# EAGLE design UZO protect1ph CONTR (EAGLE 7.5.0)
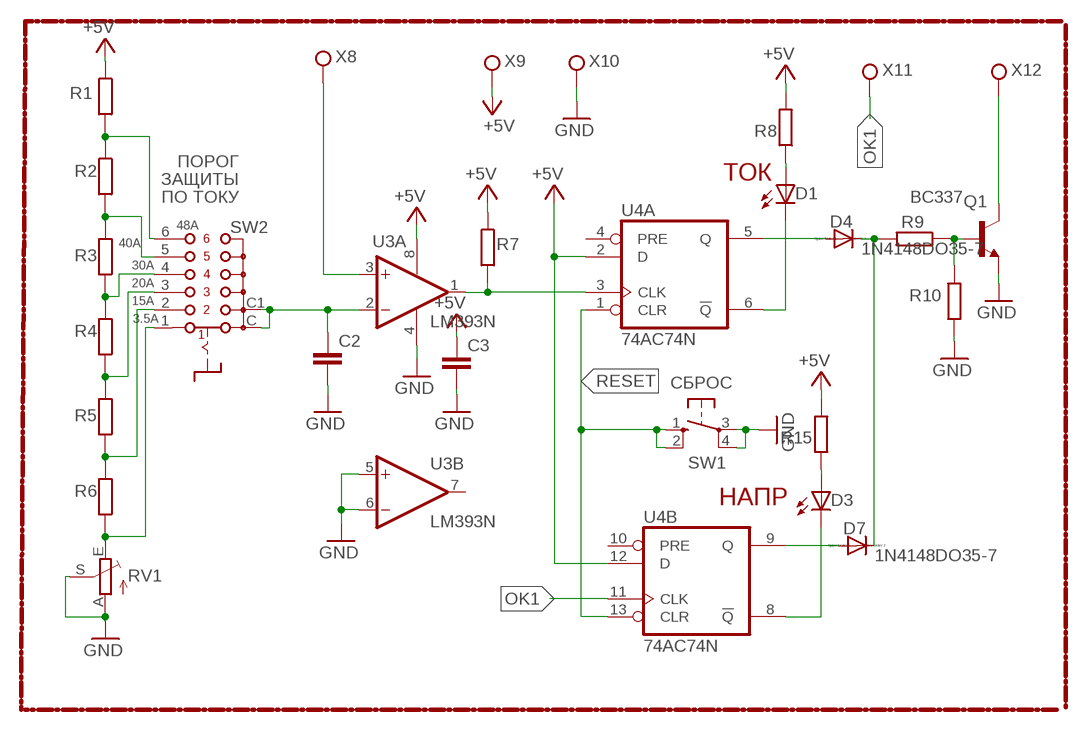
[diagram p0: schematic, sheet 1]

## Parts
C2  C-EUC1206  [C1206]
C3  C-EUC1206  [C1206]
D1  LED5MM  [LED5MM]
D3  LED5MM  [LED5MM]
D4  1N4148DO35-7  [DO35-7]
D7  1N4148DO35-7  [DO35-7]
Q1  BC337  [TO92]
R1  R-EU_R1206  [R1206]
R2  R-EU_R1206  [R1206]
R3  R-EU_R1206  [R1206]
R4  R-EU_R1206  [R1206]
R5  R-EU_R1206  [R1206]
R6  R-EU_R1206  [R1206]
R7  R-EU_R1206  [R1206]
R8  R-EU_R1206  [R1206]
R9  R-EU_R1206  [R1206]
R10  R-EU_R1206  [R1206]
R15  R-EU_R1206  [R1206]
RV1  TRIM_EU-RS3  [RS3]
SW1  SPST Push Button  10-XX  [B3F-10XX]
SW2  SS-10-16  [SS-10-16]
U3  LM393N  [DIL08]
U4  74AC74N  [DIL14]
X8  TPPAD1-17  [P1-17]
X9  TPPAD1-17  [P1-17]
X10  TPPAD1-17  [P1-17]
X11  TPPAD1-17  [P1-17]
X12  TPPAD1-17  [P1-17]

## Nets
+5V: C3.1 R1.1 R7.1 R8.2 R15.2 U3.8(P:V+) U4.2(A:D) U4.12(B:D) X9.TP
GND: C2.2 C3.2 Q1.1(E) R10.2 RV1.A RV1.S SW1.3(P) SW1.4(P1) U3.4(P:V-) U3.5(B:+IN) U3.6(B:-IN) X10.TP
N$6: U3.3(A:+IN) X8.TP
N$17: R7.2 U3.1(A:OUT) U4.3(A:CLK)
N$20: R1.2 R2.1 SW2.6
N$21: R3.1 R4.2 SW2.4
N$22: R2.2 R3.2 SW2.5
N$23: C2.1 SW2.C SW2.C1 U3.2(A:-IN)
N$24: R4.1 R5.2 SW2.3
N$25: D1.A R8.1
N$26: R5.1 R6.2 SW2.2
N$27: D3.A R15.1
N$28: Q1.2(B) R9.1 R10.1
N$29: R6.1 RV1.E SW2.1
N$30: D4.A U4.5(A:Q)
N$31: D4.C D7.C R9.2
N$32: D7.A U4.9(B:Q)
N$33: Q1.3(C) X12.TP
OK1: U4.11(B:CLK) X11.TP
PB1: D3.K(C) U4.8(B:!Q)
PB4: D1.K(C) U4.6(A:!Q)
RESET: SW1.1(S) SW1.2(S1) U4.1(A:CLR) U4.13(B:CLR)
Unconnected: U3.7(B:OUT) U4.4(A:PRE) U4.10(B:PRE)

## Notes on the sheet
- ПОРОГ
- ЗАЩИТЫ | ТОК
- ПО ТОКУ
- 48A
- 40A
- 30A
- 20A
- 15A
- 3.5A
- СБРОС
- НАПР

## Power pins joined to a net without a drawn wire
GND: U4.7(P:GND)
VCC: U4.14(P:VCC)

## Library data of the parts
C2 C3 = rcl:C-EU: CAPACITOR, European symbol
D1 D3 = led:LED: LED
D4 D7 = diode:1N4148: DIODE
Q1 = transistor:BC337: NPN TRANSISTOR
R1-R10 R15 = rcl:R-EU_: RESISTOR, European symbol
RV1 = pot:TRIM_EU-: POTENTIOMETER
SW1 = switch-omron:10-XX: OMRON SWITCH; MPN: B3F-1000; OC_FARNELL: 176432; OC_NEWARK: 36M3542
SW2 = switch:SS-10-16: Rotary Switch, Through Hole, 6 Position, 1 Pole
U3 = linear:LM393: COMPARATOR
U4 = 74xx-eu:74*74: Dual D type positive edge triggered FLIP FLOP, preset and clear
X8-X12 = testpad:TP: Test pad

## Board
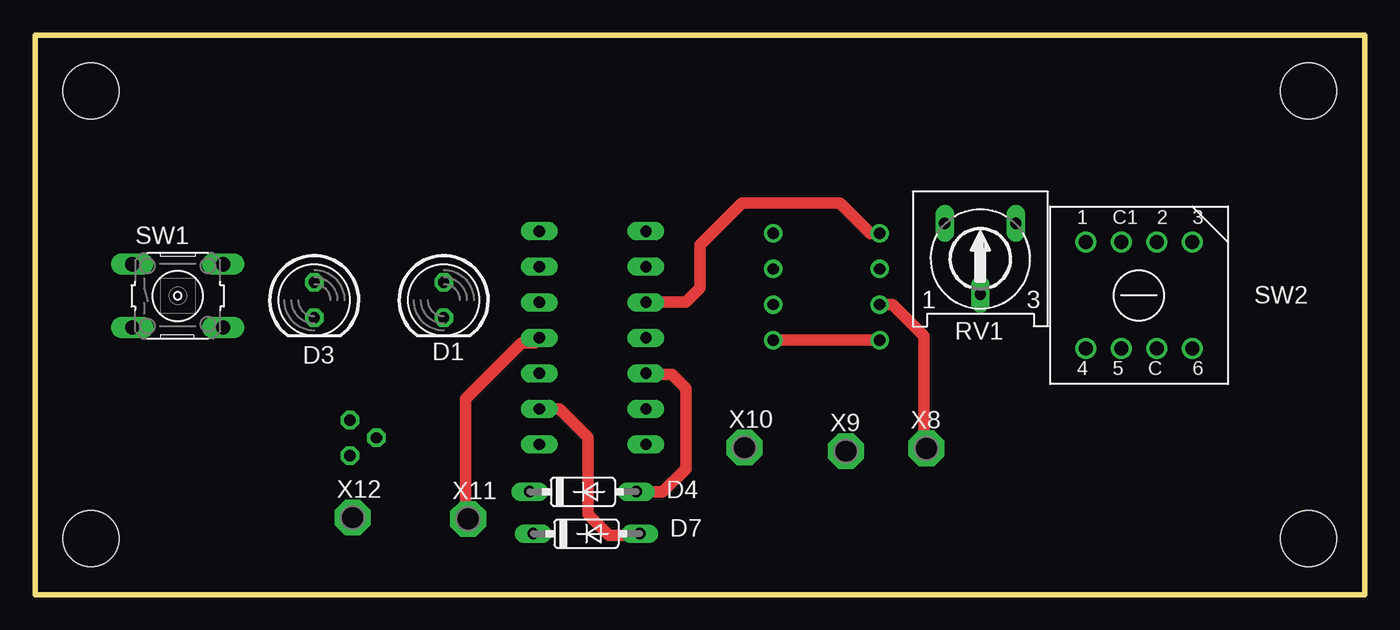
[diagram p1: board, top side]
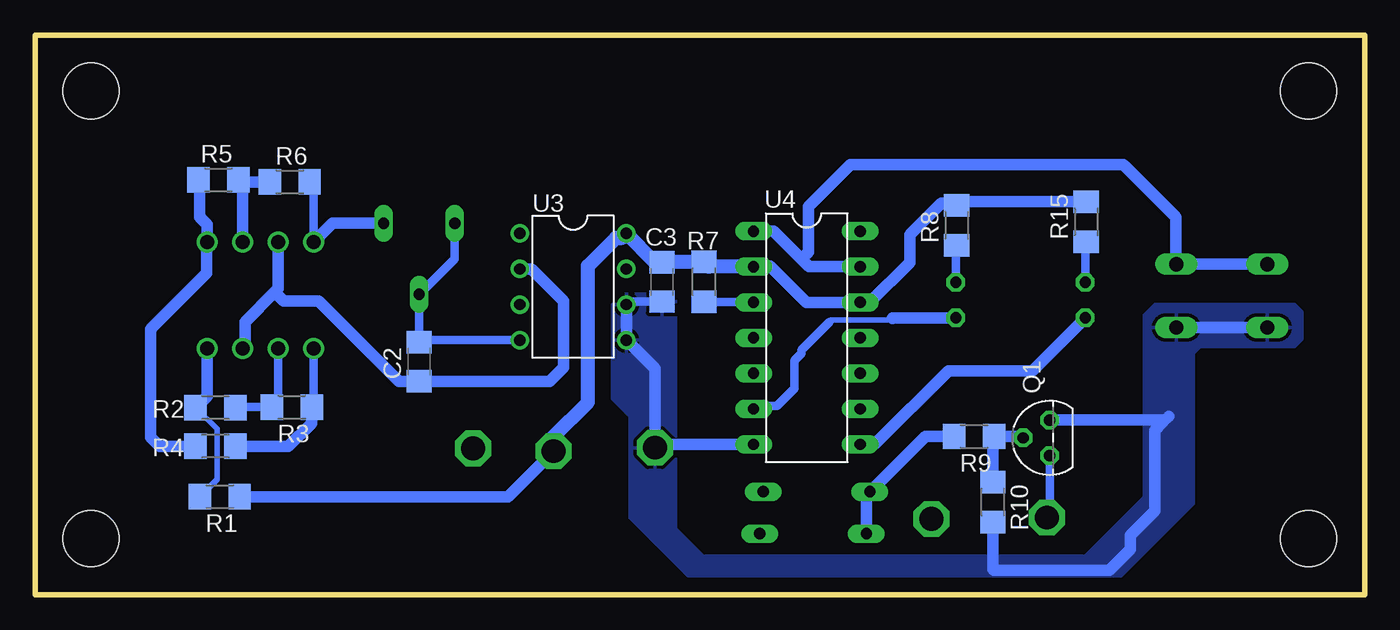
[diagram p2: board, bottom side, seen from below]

Size 95 x 40 mm. Coordinates in mm from the lower left corner, seen from the top.
Outline: 0,0 95,0 95,40 0,40 0,0
Copper layers (1*16): Top 0.035mm / dielectric 1.5mm / Bottom 0.035mm
Design rules "default": minimum track width 10mil, minimum drill 24mil, track to track 8mil, track to pad 8mil, pad to pad 8mil, via to via 8mil, smd to smd 8mil, copper to edge 40mil, drill to drill 8mil, minimum pad ring 10mil, minimum via ring 8mil, stop-mask expansion 4mil, vias tented up to drill 0mil, thermal gap 10mil
Holes 4 mm at 4,4 91,4 91,36 4,36

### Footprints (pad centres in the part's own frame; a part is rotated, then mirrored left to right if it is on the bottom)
C1206 = smd 1.6 x 1.8: 1 -1.4,0; 2 1.4,0
LED5MM = drill 0.813 octagon: A -1.27,0; K 1.27,0
DO35-7 = drill 0.813 long: A 3.81,0; C -3.81,0
TO92 = drill 0.813 octagon: 1 1.27,0; 2 0,1.905; 3 -1.27,0
R1206 = smd 1.6 x 1.803: 1 -1.422,0; 2 1.422,0
RS3 = drill 0.813 long: A -2.54,2.54; E 2.54,2.54; S 0,-2.54
B3F-10XX = drill 1.016 long: 1 -3.251,2.261; 2 3.251,2.261; 3 -3.251,-2.261; 4 3.251,-2.261
SS-10-16 = drill 1: 1 -7.62,0; 2 -2.54,0; 3 0,0; 4 -7.62,-7.62; 5 -5.08,-7.62; 6 0,-7.62; C -2.54,-7.62; C1 -5.08,0
DIL08 = drill 0.813 pad 1.27: 1 -3.81,-3.81; 2 -1.27,-3.81; 3 1.27,-3.81; 4 3.81,-3.81; 5 3.81,3.81; 6 1.27,3.81; 7 -1.27,3.81; 8 -3.81,3.81
DIL14 = drill 0.813 long: 1 -7.62,-3.81; 2 -5.08,-3.81; 3 -2.54,-3.81; 4 0,-3.81; 5 2.54,-3.81; 6 5.08,-3.81; 7 7.62,-3.81; 8 7.62,3.81; 9 5.08,3.81; 10 2.54,3.81; 11 0,3.81; 12 -2.54,3.81; 13 -5.08,3.81; 14 -7.62,3.81
P1-17 = drill 1.702 pad 2.54 octagon: TP 0,0

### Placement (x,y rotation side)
C2  67.55,16.65 90 bottom
C3  50.2,22.35 270 bottom
D1  29.2,21.05 270 top
D3  19.95,21.05 270 top
D4  39.15,7.35 0 top
D7  39.4,4.35 0 top
Q1  22.5,11.2 90 bottom
R1  81.8,7 180 bottom
R2  82.1,13.35 0 bottom
R3  76.65,13.4 180 bottom
R4  82.1,10.6 0 bottom
R5  81.9,29.65 180 bottom
R6  76.8,29.5 180 bottom
R7  47.2,22.35 270 bottom
R8  29.15,26.4 90 bottom
R9  27.9,11.3 180 bottom
R10  26.55,6.6 270 bottom
R15  19.9,26.65 90 bottom
RV1  67.55,24 0 top
SW1  10.2,21.35 0 top
SW2  82.7,25.2 0 top
U3  56.55,22 270 bottom
U4  39.85,18.35 270 bottom
X8  63.7,10.45 0 top
X9  57.95,10.25 0 top
X10  50.7,10.5 0 top
X11  30.95,5.4 0 top
X12  22.7,5.5 0 top

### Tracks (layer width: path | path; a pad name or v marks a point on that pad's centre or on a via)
+5V
  Bottom 0.813: U4.2 43.59,23.5 42.5,23.5 39.89,20.89 U4.12 35.36,20.89 32.5,23.75 32.5,25.75 30.25,28 29.33,28 R8.2 28.9,28.07 R15.2 | R1.1 61.2,7 X9.TP
  Bottom 1.016: X9.TP 57.95,11.3 55.5,13.75 55.5,23.5 53.5,25.5 53.05,25.5 U3.8 50.68,23.75 C3.1 50.18,23.77 R7.1 46.86,23.43 U4.2
GND
  Top 0.813: U3.5 U3.4
  Bottom 0.61: RV1.A 65.01,24 RV1.S C2.2 67.41,18.19 U3.4 | C3.2 50.75,20.95 52.52,20.95 U3.6
  Bottom 0.813: U3.6 U3.5 50.7,16.15 X10.TP 50.47,10.73 U4.7 | 50.47,20.67 50.75,20.95 | SW1.3 SW1.4 | R10.2 26.55,1.8 26.5,1.75 18.25,1.75 16.75,3.25 16.75,4.25 15,6 15,11.75 14.38,12.38 | 14.38,12.38 14,12.75 | Q1.1 14.47,12.47 14.38,12.38
  pour Bottom (isolate 0.813): 5,20.75 15,20.75 15.75,20 15.75,7 20,2.75 47.25,2.75 49.25,4.75 49.25,21.25 49.5,21.5 53,21.5 53.75,20.75 53.75,14 52.5,12.75 52.5,5.5 48,1 17.75,1 12.25,6.5 12.25,17.25 11.75,17.75 5,17.75 4.5,18.25 4.5,20.25
N$6
  Top 0.813: U3.3 61.27,20.73 63.5,18.5 63.5,10.65 X8.TP
N$17
  Top 0.813: U3.1 59.69,25.81 57.5,28 50.5,28 47.5,25 47.5,21.93 46.5,20.93 43.7,20.93 U4.3
  Bottom 0.61: R7.2 43.7,20.93 U4.3
N$20
  Bottom 0.406: R2.1 82,11.83 82,8.22 R1.2
  Bottom 0.813: SW2.6 82.7,14.17 R2.1
N$21
  Bottom 0.61: SW2.4 75.08,13.55 R3.1
  Bottom 0.813: R4.2 76.9,10.6 75.25,12.25 75.25,13.38 R3.1
N$22
  Bottom 0.61: SW2.5 77.62,13.85 R3.2 80.63,13.4 R2.2
N$23
  Bottom 0.813: SW2.C1 77.62,21.88 77.88,21.62 | 77.88,21.62 80,19.5 80,17.74 SW2.C | U3.2 59.52,23.27 57.25,21 57.25,16.25 58.25,15.25 C2.1 | C2.1 67.75,15.25 68,15.5 67.8,15.5 C2.1 | C2.1 69,15.25 74.75,21 77.25,21 77.88,21.62
N$24
  Bottom 0.813: R4.1 86.1,10.6 86.75,11.25 86.75,19 82.75,23 82.75,25.15 SW2.3 82.7,26.45 83.25,27 83.25,29.58 R5.2
N$25
  Bottom 0.61: D1.A 29.2,24.93 R8.1
N$26
  Bottom 0.813: R6.2 80.33,29.5 R5.1 80.16,29.33 SW2.2
N$27
  Bottom 0.61: D3.A 19.95,25.18 R15.1
N$28
  Bottom 0.813: Q1.2 24.5,11.3 R9.1 26.55,11.23 R10.1
N$29
  Bottom 0.61: SW2.1 75.08,29.2 R6.1
  Bottom 0.813: RV1.E 73.74,26.54 SW2.1
N$30
  Top 0.813: D4.A 44.85,7.35 46.5,9 46.5,14.75 45.5,15.75 43.72,15.75 U4.5
N$31
  Bottom 0.813: D7.C 35.59,7.1 D4.C 31.39,11.3 R9.2
N$32
  Top 0.813: U4.9 37.48,13.27 39.5,11.25 39.5,5.75 41,4.25 43.11,4.25 D7.A
N$33
  Bottom 0.61: Q1.3 22.5,5.7 X12.TP
OK1
  Top 0.813: X11.TP 30.75,5.6 30.75,14 34.75,18 35.69,18 U4.11
PB1
  Bottom 0.813: U4.8 35.02,10.73 29.75,16 23.73,16 D3.K
PB4
  Bottom 0.406: 33.75,19.75 34,19.75 34,19.62 38.12,19.62 38.25,19.5
  Bottom 0.61: U4.6 43.43,13.5 42,13.5 40.75,14.75 40.75,16.75 40.25,17.25 40.25,17.5 38.25,19.5
  Bottom 0.813: D1.K 33.72,19.78 33.75,19.75
RESET
  Bottom 0.813: SW1.1 SW1.2 13.5,23.66 13.5,27 17.25,30.75 36.75,30.75 39.75,27.75 39.75,24.5 40.25,24 | U4.13 39.68,23.43 40.25,24 | 40.25,24 42.25,26 43.63,26 U4.1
